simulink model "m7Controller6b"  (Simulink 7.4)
settings: Solver=FixedStepDiscrete  StartTime=0.0  StopTime=100  FixedStep=0.1  RelTol=1e-3
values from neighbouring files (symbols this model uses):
  Link1 = [pi/2, 0, pi/2, 0]    [robot_parameters.m]
  Link2 = [0, 0.404, pi/2, 0]    [robot_parameters.m]
  Link3 = [-pi/2, 0, 0, 0]    [robot_parameters.m]
  Link4 = [pi/2, 0.025, 0, 0.405]    [robot_parameters.m]
  Link5 = [pi/2, 0, pi/2, 0]    [robot_parameters.m]
  Link6 = [0, 0, pi/2, 0]    [robot_parameters.m]
  NoOfLinks = 6    [robot_parameters.m]
libraries: vrlib x3, simulink x2

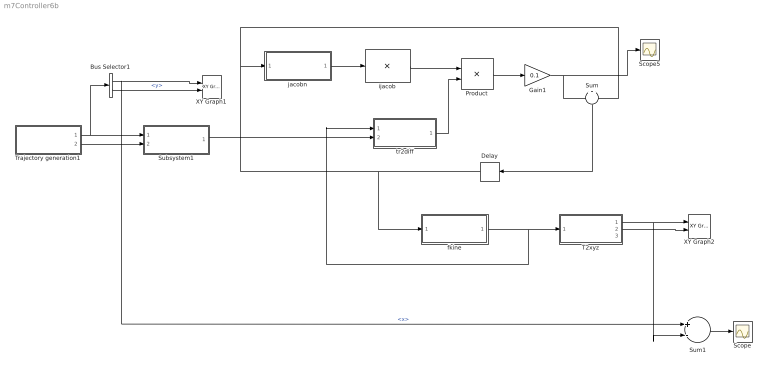
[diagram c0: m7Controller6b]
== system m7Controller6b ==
  Bus Selector1 : BusSelector  OutputSignals=x,y
  Delay : Memory  X0=[pi/2; pi/2; 0; 0; pi/2; pi/2]  InheritSampleTime=on
  Gain1 : Gain  Gain=0.1  ParameterDataType=fixdt(1, 16)  ParameterScaling=2^0  OutDataType=fixdt(1, 16)  OutScaling=2^0
  Product : Product  Multiplication=Matrix(*)  OutDataType=sfix(16)  OutScaling=2^0
  Scope : Scope
  Scope5 : Scope
  Subsystem1 : Subsystem
  Sum : Sum  OutDataType=sfix(16)  OutScaling=2^0
  Sum1 : Sum  Inputs=+-  OutDataType=sfix(16)  OutScaling=2^0
  T2xyz : Subsystem
  Trajectory generation1 : Subsystem
  XY Graph1 : simulink/Sinks/XY Graph  SystemSampleTime=-1  xmin=-0.2  xmax=0.8  ymin=-0.5  ymax=0.5  st=-1
  XY Graph2 : simulink/Sinks/XY Graph  SystemSampleTime=-1  xmin=-0.2  xmax=0.8  ymin=-0.5  ymax=0.5  st=-1
  fkine : Subsystem  TreatAsAtomicUnit=on
  ijacob : Product  Inputs=/  Multiplication=Matrix(*)  OutDataType=fixdt(1, 16)  OutScaling=2^0
  jacobn : Subsystem  TreatAsAtomicUnit=on
  tr2diff : Subsystem
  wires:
  T2xyz/1(x) -> Sum1/2, XY Graph2/1
  fkine/1(T) -> T2xyz/1(T), tr2diff/1(T1)
  jacobn/1(Out1) -> ijacob/1
  ijacob/1 -> Product/1
  Sum/1 -> Delay/1
  Delay/1 -> Sum/2, jacobn/1(q), fkine/1(q)
  Trajectory generation1/1(xyz) -> Subsystem1/1(xyz), Bus Selector1/1
  Trajectory generation1/2(rpy) -> Subsystem1/2(rpy)
  Bus Selector1/1 -> Sum1/1, XY Graph1/1  "<x>"
  Subsystem1/1(T) -> tr2diff/2(T2)
  Product/1 -> Gain1/1
  Gain1/1 -> Scope5/1, Sum/1
  Sum1/1 -> Scope/1
  Bus Selector1/2 -> XY Graph1/2  "<y>"
  T2xyz/2(y) -> XY Graph2/2
  tr2diff/1(dx) -> Product/2

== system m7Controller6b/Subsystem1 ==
  xyz : Inport  OutDataType=fixdt(1, 16)  OutScaling=2^0
  rpy : Inport  Port=2  OutDataType=fixdt(1, 16)  OutScaling=2^0
  Bus Selector : BusSelector  OutputSignals=x,y,z
  Bus Selector1 : BusSelector  OutputSignals=roll,pitch,yaw
  Product : Product  Multiplication=Matrix(*)  OutDataType=fixdt(1, 16)  OutScaling=2^0
  rpy2T : Subsystem
  xyz2T : Subsystem
  T : Outport  OutDataType=fixdt(1, 16)  OutScaling=2^0
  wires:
  xyz/1 -> Bus Selector/1
  Bus Selector/1 -> xyz2T/1(x)  "<x>"
  Bus Selector/2 -> xyz2T/2(y)  "<y>"
  Bus Selector/3 -> xyz2T/3(z)  "<z>"
  xyz2T/1(T) -> Product/1
  Product/1 -> T/1
  rpy2T/1(T) -> Product/2
  rpy/1 -> Bus Selector1/1
  Bus Selector1/1 -> rpy2T/1(roll)  "<roll>"
  Bus Selector1/2 -> rpy2T/2(pitch)  "<pitch>"
  Bus Selector1/3 -> rpy2T/3(yaw)  "<yaw>"

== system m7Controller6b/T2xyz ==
  T : Inport  OutDataType=fixdt(1, 16)  OutScaling=2^0
  Selector : Selector  NumberOfDimensions=2  InputPortWidth=3  IndexOptions=Index vector (dialog),Index vector (dialog)  Indices=1,4  OutputSizes=1,1
  Selector1 : Selector  NumberOfDimensions=2  InputPortWidth=3  IndexOptions=Index vector (dialog),Index vector (dialog)  Indices=2,4  OutputSizes=1,1
  Selector2 : Selector  NumberOfDimensions=2  InputPortWidth=3  IndexOptions=Index vector (dialog),Index vector (dialog)  Indices=3,4  OutputSizes=1,1
  x : Outport  OutDataType=fixdt(1, 16)  OutScaling=2^0
  y : Outport  Port=2  OutDataType=fixdt(1, 16)  OutScaling=2^0
  z : Outport  Port=3  OutDataType=fixdt(1, 16)  OutScaling=2^0
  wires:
  Selector/1 -> x/1
  Selector1/1 -> y/1
  Selector2/1 -> z/1
  T/1 -> Selector/1, Selector2/1, Selector1/1

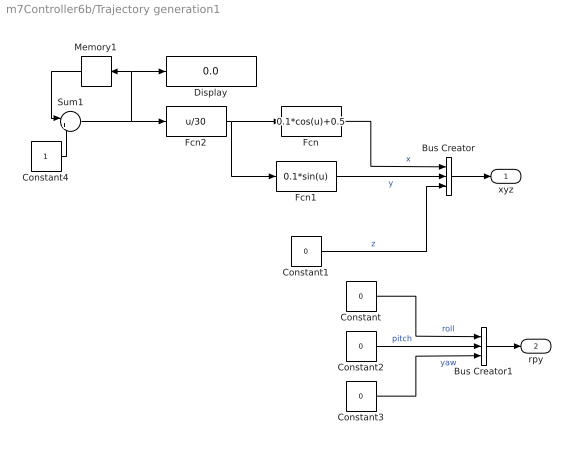
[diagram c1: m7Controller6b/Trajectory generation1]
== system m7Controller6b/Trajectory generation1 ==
  Bus Creator : BusCreator  Inputs='x','y','z'
  Bus Creator1 : BusCreator  Inputs=3
  Constant : Constant  Value=0  VectorParams1D=off  OutDataType=fixdt(1, 16)  OutScaling=2^0
  Constant1 : Constant  Value=0
  Constant2 : Constant  Value=0  OutDataType=fixdt(1, 16)  OutScaling=2^0
  Constant3 : Constant  Value=0  OutDataType=fixdt(1, 16)  OutScaling=2^0
  Constant4 : Constant  OutDataType=fixdt(1, 16)  OutScaling=2^0
  Display : Display
  Fcn : Fcn  Expr=0.1*cos(u)+0.5
  Fcn1 : Fcn  Expr=0.1*sin(u)
  Fcn2 : Fcn  Expr=u/30
  Memory1 : Memory
  Sum1 : Sum  Inputs=|++  OutDataType=sfix(16)  OutScaling=2^0
  xyz : Outport  OutDataType=fixdt(1, 16)  OutScaling=2^0
  rpy : Outport  Port=2  OutDataType=fixdt(1, 16)  OutScaling=2^0
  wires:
  Constant1/1 -> Bus Creator/3  "z"
  Fcn2/1 -> Fcn/1, Fcn1/1
  Fcn/1 -> Bus Creator/1  "x"
  Fcn1/1 -> Bus Creator/2  "y"
  Bus Creator/1 -> xyz/1
  Constant2/1 -> Bus Creator1/2  "pitch"
  Constant/1 -> Bus Creator1/1  "roll"
  Constant3/1 -> Bus Creator1/3  "yaw"
  Bus Creator1/1 -> rpy/1
  Memory1/1 -> Sum1/1
  Sum1/1 -> Fcn2/1, Display/1, Memory1/1
  Constant4/1 -> Sum1/2

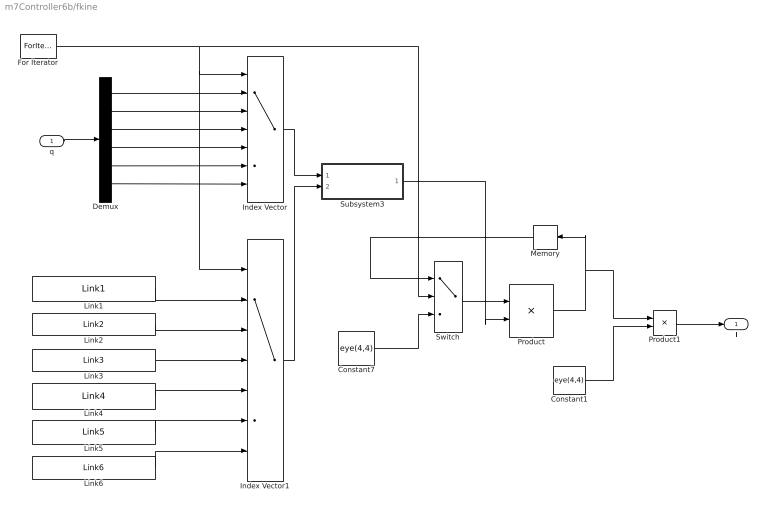
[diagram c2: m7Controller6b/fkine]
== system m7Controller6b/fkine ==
  q : Inport  OutDataType=fixdt(1, 16)  OutScaling=2^0
  Constant1 : Constant  Value=eye(4,4)  OutDataType=fixdt(1, 16)  OutScaling=2^0
  Constant7 : Constant  Value=eye(4,4)  OutDataType=fixdt(1, 16)  OutScaling=2^0
  Demux : Demux  Outputs=6
  For Iterator : ForIterator  IterationLimit=NoOfLinks
  Index Vector : MultiPortSwitch  Inputs=6  OutDataType=fixdt(1, 16)  OutScaling=2^0
  Index Vector1 : MultiPortSwitch  Inputs=6  OutDataType=fixdt(1, 16)  OutScaling=2^0
  Link1 : Constant  Value=Link1  OutDataType=fixdt(1, 16)  OutScaling=2^0
  Link2 : Constant  Value=Link2  OutDataType=fixdt(1, 16)  OutScaling=2^0
  Link3 : Constant  Value=Link3  OutDataType=fixdt(1, 16)  OutScaling=2^0
  Link4 : Constant  Value=Link4  OutDataType=fixdt(1, 16)  OutScaling=2^0
  Link5 : Constant  Value=Link5  OutDataType=fixdt(1, 16)  OutScaling=2^0
  Link6 : Constant  Value=Link6  OutDataType=fixdt(1, 16)  OutScaling=2^0
  Memory : Memory  X0=eye(4,4)  InheritSampleTime=on
  Product : Product  Multiplication=Matrix(*)  OutDataType=fixdt(1, 16)  OutScaling=2^0
  Product1 : Product  Multiplication=Matrix(*)  OutDataType=fixdt(1,8,2)
  Subsystem3 : Subsystem
  Switch : Switch  Criteria=u2 > Threshold  Threshold=1  OutDataType=fixdt(1, 16)  OutScaling=2^0
  T : Outport  OutDataType=fixdt(1, 16)  OutScaling=2^0
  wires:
  Memory/1 -> Switch/1
  Switch/1 -> Product/1
  Subsystem3/1(Out1) -> Product/2
  Constant7/1 -> Switch/3
  Product/1 -> Product1/1, Memory/1
  Index Vector1/1 -> Subsystem3/2(In2)
  Index Vector/1 -> Subsystem3/1(In1)
  Demux/6 -> Index Vector/7
  Demux/5 -> Index Vector/6
  Demux/4 -> Index Vector/5
  Demux/3 -> Index Vector/4
  Demux/2 -> Index Vector/3
  Demux/1 -> Index Vector/2
  q/1 -> Demux/1
  Link6/1 -> Index Vector1/7
  Link5/1 -> Index Vector1/6
  Link4/1 -> Index Vector1/5
  Link3/1 -> Index Vector1/4
  Link2/1 -> Index Vector1/3
  Link1/1 -> Index Vector1/2
  For Iterator/1 -> Switch/2, Index Vector1/1, Index Vector/1
  Product1/1 -> T/1
  Constant1/1 -> Product1/2

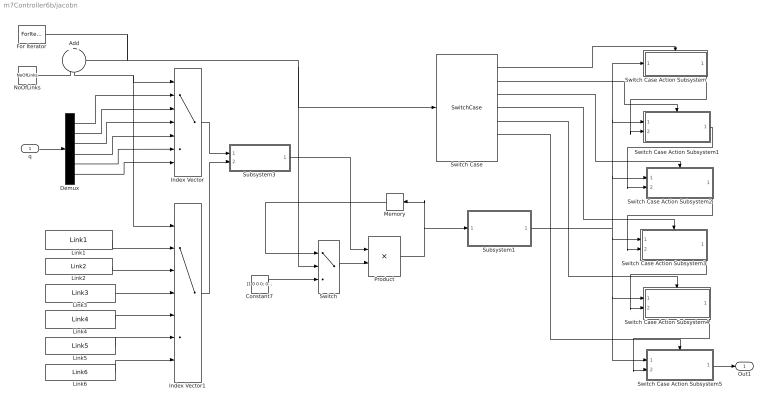
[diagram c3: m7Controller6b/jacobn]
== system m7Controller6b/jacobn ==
  q : Inport  OutDataType=fixdt(1, 16)  OutScaling=2^0
  Add : Sum  Inputs=+-  OutDataType=fixdt(1, 16)  OutScaling=2^-10
  Constant7 : Constant  Value=[1 0 0 0; 0 1 0 0; 0 0 1 0; 0 0 0 1]  OutDataType=fixdt(1, 16)  OutScaling=2^0
  Demux : Demux  Outputs=6
  For Iterator : ForIterator  IterationLimit=NoOfLinks
  Index Vector : MultiPortSwitch  Inputs=6  zeroidx=on  OutDataType=fixdt(1, 16)  OutScaling=2^0
  Index Vector1 : MultiPortSwitch  Inputs=6  zeroidx=on  OutDataType=fixdt(1, 16)  OutScaling=2^0
  Link1 : Constant  Value=Link1  OutDataType=fixdt(1, 16)  OutScaling=2^0
  Link2 : Constant  Value=Link2  OutDataType=fixdt(1, 16)  OutScaling=2^0
  Link3 : Constant  Value=Link3  OutDataType=fixdt(1, 16)  OutScaling=2^0
  Link4 : Constant  Value=Link4  OutDataType=fixdt(1, 16)  OutScaling=2^0
  Link5 : Constant  Value=Link5  OutDataType=fixdt(1, 16)  OutScaling=2^0
  Link6 : Constant  Value=Link6  OutDataType=fixdt(1, 16)  OutScaling=2^0
  Memory : Memory  X0=[1 0 0 0; 0 1 0 0; 0 0 1 0; 0 0 0 1]  InheritSampleTime=on
  NoOfLinks : Constant  Value=NoOfLinks  OutDataType=fixdt(1, 16)  OutScaling=2^0
  Product : Product  Multiplication=Matrix(*)  OutDataType=fixdt(1, 16)  OutScaling=2^0
  Subsystem1 : Subsystem
  Subsystem3 : Subsystem
  Switch : Switch  Threshold=1  OutDataType=fixdt(1, 16)  OutScaling=2^0
  Switch Case : SwitchCase  CaseConditions={1, 2, 3, 4, 5, 6}
  Switch Case Action Subsystem : Subsystem  TreatAsAtomicUnit=on
  Switch Case Action Subsystem1 : Subsystem  TreatAsAtomicUnit=on
  Switch Case Action Subsystem2 : Subsystem  TreatAsAtomicUnit=on
  Switch Case Action Subsystem3 : Subsystem  TreatAsAtomicUnit=on
  Switch Case Action Subsystem4 : Subsystem  TreatAsAtomicUnit=on
  Switch Case Action Subsystem5 : Subsystem  TreatAsAtomicUnit=on
  Out1 : Outport  OutDataType=fixdt(1, 16)  OutScaling=2^0
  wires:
  NoOfLinks/1 -> Add/1
  For Iterator/1 -> Add/2, Switch/2, Switch Case/1
  Add/1 -> Index Vector/1, Index Vector1/1
  Link1/1 -> Index Vector1/2
  Link2/1 -> Index Vector1/3
  Link3/1 -> Index Vector1/4
  Link4/1 -> Index Vector1/5
  Link5/1 -> Index Vector1/6
  Link6/1 -> Index Vector1/7
  q/1 -> Demux/1
  Demux/1 -> Index Vector/2
  Demux/2 -> Index Vector/3
  Demux/3 -> Index Vector/4
  Demux/4 -> Index Vector/5
  Demux/5 -> Index Vector/6
  Demux/6 -> Index Vector/7
  Index Vector/1 -> Subsystem3/1(In1)
  Index Vector1/1 -> Subsystem3/2(In2)
  Product/1 -> Memory/1, Subsystem1/1(In1)
  Constant7/1 -> Switch/3
  Subsystem3/1(Out1) -> Product/1
  Switch/1 -> Product/2
  Memory/1 -> Switch/1
  Subsystem1/1(Out1) -> Switch Case Action Subsystem/1(In1), Switch Case Action Subsystem1/1(In1), Switch Case Action Subsystem2/1(In1), Switch Case Action Subsystem5/1(In1), Switch Case Action Subsystem4/1(In1), Switch Case Action Subsystem3/1(In1)
  Switch Case/1 -> Switch Case Action Subsystem/Action
  Switch Case/2 -> Switch Case Action Subsystem1/Action
  Switch Case/3 -> Switch Case Action Subsystem2/Action
  Switch Case/4 -> Switch Case Action Subsystem3/Action
  Switch Case/5 -> Switch Case Action Subsystem4/Action
  Switch Case/6 -> Switch Case Action Subsystem5/Action
  Switch Case Action Subsystem5/1(Out1) -> Out1/1
  Switch Case Action Subsystem1/1(Out1) -> Switch Case Action Subsystem2/2(In2)
  Switch Case Action Subsystem/1(Out1) -> Switch Case Action Subsystem1/2(In2)
  Switch Case Action Subsystem2/1(Out1) -> Switch Case Action Subsystem3/2(In2)
  Switch Case Action Subsystem3/1(Out1) -> Switch Case Action Subsystem4/2(In2)
  Switch Case Action Subsystem4/1(Out1) -> Switch Case Action Subsystem5/2(In2)

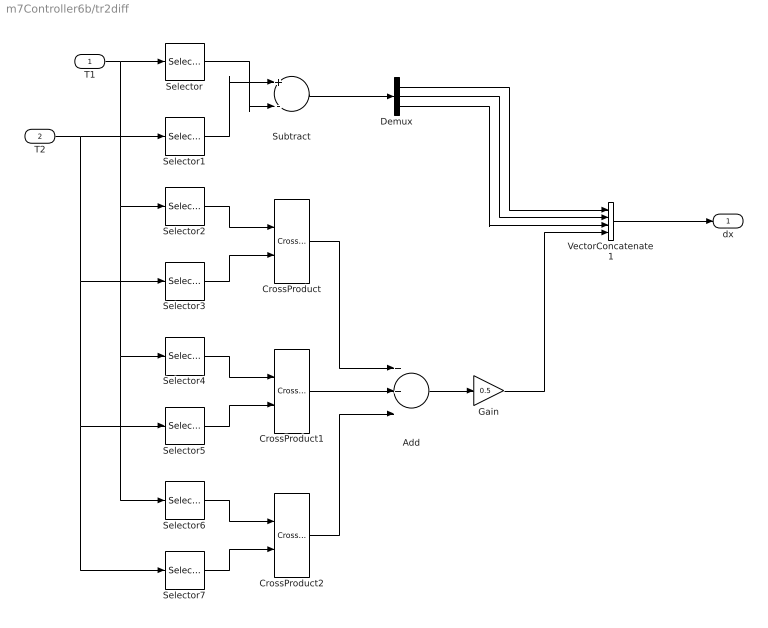
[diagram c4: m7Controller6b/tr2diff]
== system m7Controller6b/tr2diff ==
  T1 : Inport  OutDataType=fixdt(1, 16)  OutScaling=2^0
  T2 : Inport  Port=2  OutDataType=fixdt(1, 16)  OutScaling=2^0
  Add : Sum  Inputs=+++  OutDataType=fixdt(1, 16)  OutScaling=2^-10
  CrossProduct : vrlib/Utilities/Cross Product  SystemSampleTime=-1
  CrossProduct1 : vrlib/Utilities/Cross Product  SystemSampleTime=-1
  CrossProduct2 : vrlib/Utilities/Cross Product  SystemSampleTime=-1
  Demux : Demux  Outputs=3
  Gain : Gain  Gain=0.5  ParameterDataType=fixdt(1, 16)  ParameterScaling=2^0  OutDataType=fixdt(1, 16)  OutScaling=2^0
  Selector : Selector  NumberOfDimensions=2  InputPortWidth=3  IndexOptions=Index vector (dialog),Index vector (dialog)  Indices=[1:3],4  OutputSizes=1,1
  Selector1 : Selector  NumberOfDimensions=2  InputPortWidth=3  IndexOptions=Index vector (dialog),Index vector (dialog)  Indices=[1:3],4  OutputSizes=1,1
  Selector2 : Selector  NumberOfDimensions=2  InputPortWidth=3  IndexOptions=Index vector (dialog),Index vector (dialog)  Indices=[1:3],1  OutputSizes=1,1
  Selector3 : Selector  NumberOfDimensions=2  InputPortWidth=3  IndexOptions=Index vector (dialog),Index vector (dialog)  Indices=[1:3],1  OutputSizes=1,1
  Selector4 : Selector  NumberOfDimensions=2  InputPortWidth=3  IndexOptions=Index vector (dialog),Index vector (dialog)  Indices=[1:3],2  OutputSizes=1,1
  Selector5 : Selector  NumberOfDimensions=2  InputPortWidth=3  IndexOptions=Index vector (dialog),Index vector (dialog)  Indices=[1:3],2  OutputSizes=1,1
  Selector6 : Selector  NumberOfDimensions=2  InputPortWidth=3  IndexOptions=Index vector (dialog),Index vector (dialog)  Indices=[1:3],3  OutputSizes=1,1
  Selector7 : Selector  NumberOfDimensions=2  InputPortWidth=3  IndexOptions=Index vector (dialog),Index vector (dialog)  Indices=[1:3],3  OutputSizes=1,1
  Subtract : Sum  Inputs=+-  OutDataType=fixdt(1, 16)  OutScaling=2^-10
  VectorConcatenate1 : Concatenate  NumInputs=4  Mode=Vector
  dx : Outport  OutDataType=fixdt(1, 16)  OutScaling=2^0
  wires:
  T1/1 -> Selector/1, Selector2/1, Selector6/1, Selector4/1
  T2/1 -> Selector1/1, Selector7/1, Selector5/1, Selector3/1
  Selector1/1 -> Subtract/1
  Selector/1 -> Subtract/2
  Selector2/1 -> CrossProduct/1
  Selector3/1 -> CrossProduct/2
  Selector4/1 -> CrossProduct1/1
  Selector5/1 -> CrossProduct1/2
  Selector6/1 -> CrossProduct2/1
  Selector7/1 -> CrossProduct2/2
  CrossProduct/1 -> Add/1
  CrossProduct1/1 -> Add/2
  CrossProduct2/1 -> Add/3
  Add/1 -> Gain/1
  VectorConcatenate1/1 -> dx/1
  Subtract/1 -> Demux/1
  Demux/1 -> VectorConcatenate1/1
  Demux/2 -> VectorConcatenate1/2
  Demux/3 -> VectorConcatenate1/3
  Gain/1 -> VectorConcatenate1/4

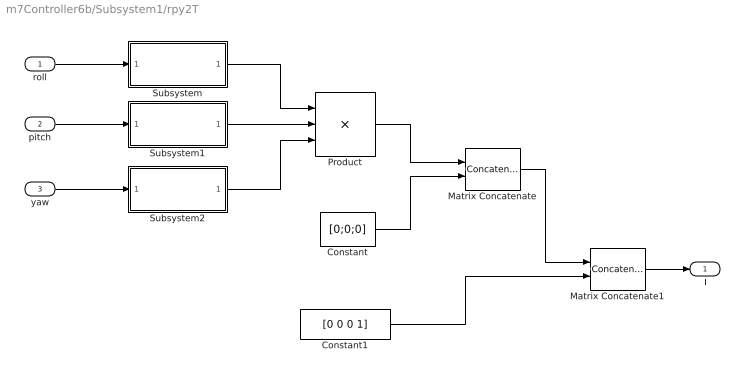
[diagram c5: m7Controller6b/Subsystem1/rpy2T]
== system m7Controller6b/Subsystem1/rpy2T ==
  roll : Inport  OutDataType=fixdt(1, 16)  OutScaling=2^0
  pitch : Inport  Port=2  OutDataType=fixdt(1, 16)  OutScaling=2^0
  yaw : Inport  Port=3  OutDataType=fixdt(1, 16)  OutScaling=2^0
  Constant : Constant  Value=[0;0;0]  OutDataType=fixdt(1, 16)  OutScaling=2^0
  Constant1 : Constant  Value=[0 0 0 1]  VectorParams1D=off  OutDataType=fixdt(1, 16)  OutScaling=2^0
  Matrix Concatenate : Concatenate  Mode=Multidimensional array  ConcatenateDimension=2
  Matrix Concatenate1 : Concatenate  Mode=Multidimensional array
  Product : Product  Inputs=3  Multiplication=Matrix(*)  OutDataType=fixdt(1, 16)  OutScaling=2^0
  Subsystem : Subsystem
  Subsystem1 : Subsystem
  Subsystem2 : Subsystem
  T : Outport  OutDataType=fixdt(1, 16)  OutScaling=2^0
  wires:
  roll/1 -> Subsystem/1(roll)
  pitch/1 -> Subsystem1/1(roll)
  yaw/1 -> Subsystem2/1(roll)
  Subsystem/1(Out1) -> Product/1
  Subsystem1/1(Out1) -> Product/2
  Subsystem2/1(Out1) -> Product/3
  Product/1 -> Matrix Concatenate/1
  Constant/1 -> Matrix Concatenate/2
  Matrix Concatenate/1 -> Matrix Concatenate1/1
  Constant1/1 -> Matrix Concatenate1/2
  Matrix Concatenate1/1 -> T/1

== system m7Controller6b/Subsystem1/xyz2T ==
  x : Inport  OutDataType=fixdt(1, 16)  OutScaling=2^0
  y : Inport  Port=2  OutDataType=fixdt(1, 16)  OutScaling=2^0
  z : Inport  Port=3  OutDataType=fixdt(1, 16)  OutScaling=2^0
  Constant : Constant  Value=eye(3)  OutDataType=fixdt(1, 16)  OutScaling=2^0
  Constant1 : Constant  Value=[0 0 0 1]  VectorParams1D=off  OutDataType=fixdt(1, 16)  OutScaling=2^0
  Matrix Concatenate : Concatenate  Mode=Multidimensional array  ConcatenateDimension=2
  Matrix Concatenate1 : Concatenate  Mode=Multidimensional array
  Vector Concatenate : Concatenate  NumInputs=3  Mode=Vector
  T : Outport  OutDataType=fixdt(1, 16)  OutScaling=2^0
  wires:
  x/1 -> Vector Concatenate/1
  y/1 -> Vector Concatenate/2
  z/1 -> Vector Concatenate/3
  Constant/1 -> Matrix Concatenate/1
  Vector Concatenate/1 -> Matrix Concatenate/2
  Matrix Concatenate/1 -> Matrix Concatenate1/1
  Constant1/1 -> Matrix Concatenate1/2
  Matrix Concatenate1/1 -> T/1

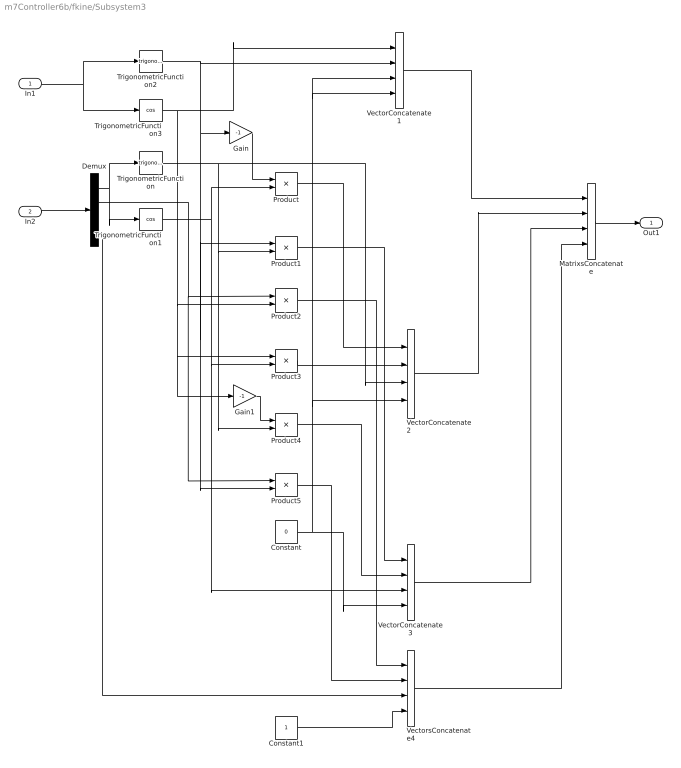
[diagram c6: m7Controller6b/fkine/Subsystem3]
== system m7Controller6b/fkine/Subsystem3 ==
  In1 : Inport  OutDataType=fixdt(1, 16)  OutScaling=2^0
  In2 : Inport  Port=2  OutDataType=fixdt(1, 16)  OutScaling=2^0
  Constant : Constant  Value=0  OutDataType=fixdt(1, 16)  OutScaling=2^0
  Constant1 : Constant  OutDataType=fixdt(1, 16)  OutScaling=2^0
  Demux : Demux
  Gain : Gain  Gain=-1  ParameterDataType=fixdt(1, 16)  ParameterScaling=2^0  OutDataType=fixdt(1, 16)  OutScaling=2^0
  Gain1 : Gain  Gain=-1  ParameterDataType=fixdt(1, 16)  ParameterScaling=2^0  OutDataType=fixdt(1, 16)  OutScaling=2^0
  MatrixsConcatenate : Concatenate  NumInputs=4  Mode=Multidimensional array  ConcatenateDimension=2
  Product{,1..5} (6 alike) : Product  OutDataType=fixdt(1, 16)  OutScaling=2^0
  TrigonometricFunction : Trigonometry
  TrigonometricFunction1 : Trigonometry  Operator=cos
  TrigonometricFunction2 : Trigonometry
  TrigonometricFunction3 : Trigonometry  Operator=cos
  VectorConcatenate1 : Concatenate  NumInputs=4  Mode=Vector  ConcatenateDimension=2
  VectorConcatenate2 : Concatenate  NumInputs=4  Mode=Vector  ConcatenateDimension=2
  VectorConcatenate3 : Concatenate  NumInputs=4  Mode=Vector  ConcatenateDimension=2
  VectorsConcatenate4 : Concatenate  NumInputs=4  Mode=Vector  ConcatenateDimension=2
  Out1 : Outport  OutDataType=fixdt(1, 16)  OutScaling=2^0
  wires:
  VectorsConcatenate4/1 -> MatrixsConcatenate/4
  VectorConcatenate3/1 -> MatrixsConcatenate/3
  VectorConcatenate2/1 -> MatrixsConcatenate/2
  VectorConcatenate1/1 -> MatrixsConcatenate/1
  MatrixsConcatenate/1 -> Out1/1
  Constant1/1 -> VectorsConcatenate4/4
  Constant/1 -> VectorConcatenate1/3, VectorConcatenate1/4, VectorConcatenate2/4, VectorConcatenate3/4
  Gain1/1 -> Product4/1
  Product3/1 -> VectorConcatenate2/2
  Demux/2 -> Product5/1, Product2/1
  TrigonometricFunction/1 -> Product1/2, Product4/2, VectorConcatenate2/3
  TrigonometricFunction3/1 -> VectorConcatenate1/1, Gain1/1, Product3/1, Product2/2
  TrigonometricFunction1/1 -> VectorConcatenate3/3, Product3/2, Product/2
  Gain/1 -> Product/1
  TrigonometricFunction2/1 -> Product1/1, Product5/2, Gain/1, VectorConcatenate1/2
  Demux/1 -> TrigonometricFunction1/1, TrigonometricFunction/1
  In1/1 -> TrigonometricFunction3/1, TrigonometricFunction2/1
  In2/1 -> Demux/1
  Product/1 -> VectorConcatenate2/1
  Product4/1 -> VectorConcatenate3/2
  Product1/1 -> VectorConcatenate3/1
  Product2/1 -> VectorsConcatenate4/1
  Product5/1 -> VectorsConcatenate4/2
  Demux/4 -> VectorsConcatenate4/3

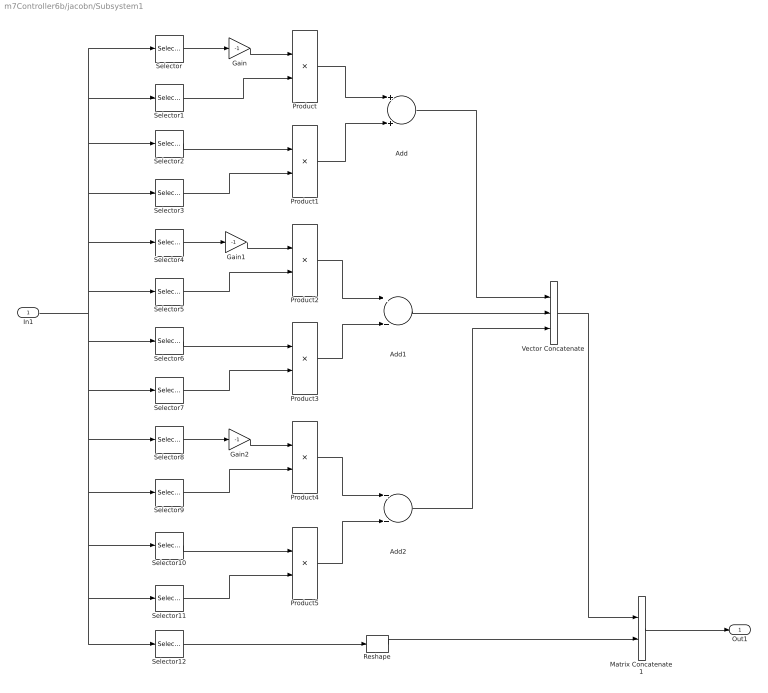
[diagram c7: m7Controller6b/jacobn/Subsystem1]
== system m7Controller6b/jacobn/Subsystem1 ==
  In1 : Inport
  Add : Sum  OutDataType=fixdt(1, 16)  OutScaling=2^-10
  Add1 : Sum  OutDataType=fixdt(1, 16)  OutScaling=2^-10
  Add2 : Sum  OutDataType=fixdt(1, 16)  OutScaling=2^-10
  Gain : Gain  Gain=-1  ParameterDataType=fixdt(1, 16)  ParameterScaling=2^0  OutDataType=fixdt(1, 16)  OutScaling=2^0
  Gain1 : Gain  Gain=-1  ParameterDataType=fixdt(1, 16)  ParameterScaling=2^0  OutDataType=fixdt(1, 16)  OutScaling=2^0
  Gain2 : Gain  Gain=-1  ParameterDataType=fixdt(1, 16)  ParameterScaling=2^0  OutDataType=fixdt(1, 16)  OutScaling=2^0
  Matrix Concatenate1 : Concatenate  Mode=Multidimensional array
  Product{,1..5} (6 alike) : Product  OutDataType=fixdt(1, 16)  OutScaling=2^0
  Reshape : Reshape  OutputDimensionality=Customize  OutputDimensions=[3,1]
  Selector : Selector  NumberOfDimensions=2  InputPortWidth=3  IndexOptions=Index vector (dialog),Index vector (dialog)  Indices=1,1  OutputSizes=1,1
  Selector1 : Selector  NumberOfDimensions=2  InputPortWidth=3  IndexOptions=Index vector (dialog),Index vector (dialog)  Indices=2,4  OutputSizes=1,1
  Selector10 : Selector  NumberOfDimensions=2  InputPortWidth=3  IndexOptions=Index vector (dialog),Index vector (dialog)  Indices=2,3  OutputSizes=1,1
  Selector11 : Selector  NumberOfDimensions=2  InputPortWidth=3  IndexOptions=Index vector (dialog),Index vector (dialog)  Indices=1,4  OutputSizes=1,1
  Selector12 : Selector  NumberOfDimensions=2  InputPortWidth=3  IndexOptions=Index vector (dialog),Index vector (dialog)  Indices=3,[1:3]  OutputSizes=1,1
  Selector2 : Selector  NumberOfDimensions=2  InputPortWidth=3  IndexOptions=Index vector (dialog),Index vector (dialog)  Indices=2,1  OutputSizes=1,1
  Selector3 : Selector  NumberOfDimensions=2  InputPortWidth=3  IndexOptions=Index vector (dialog),Index vector (dialog)  Indices=1,4  OutputSizes=1,1
  Selector4 : Selector  NumberOfDimensions=2  InputPortWidth=3  IndexOptions=Index vector (dialog),Index vector (dialog)  Indices=1,2  OutputSizes=1,1
  Selector5 : Selector  NumberOfDimensions=2  InputPortWidth=3  IndexOptions=Index vector (dialog),Index vector (dialog)  Indices=2,4  OutputSizes=1,1
  Selector6 : Selector  NumberOfDimensions=2  InputPortWidth=3  IndexOptions=Index vector (dialog),Index vector (dialog)  Indices=2,2  OutputSizes=1,1
  Selector7 : Selector  NumberOfDimensions=2  InputPortWidth=3  IndexOptions=Index vector (dialog),Index vector (dialog)  Indices=1,4  OutputSizes=1,1
  Selector8 : Selector  NumberOfDimensions=2  InputPortWidth=3  IndexOptions=Index vector (dialog),Index vector (dialog)  Indices=1,3  OutputSizes=1,1
  Selector9 : Selector  NumberOfDimensions=2  InputPortWidth=3  IndexOptions=Index vector (dialog),Index vector (dialog)  Indices=2,4  OutputSizes=1,1
  Vector Concatenate : Concatenate  NumInputs=3  Mode=Vector
  Out1 : Outport
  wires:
  Selector/1 -> Gain/1
  In1/1 -> Selector/1, Selector1/1, Selector2/1, Selector3/1, Selector4/1, Selector5/1, Selector10/1, Selector11/1, Selector12/1, Selector9/1, Selector8/1, Selector7/1, Selector6/1
  Gain/1 -> Product/1
  Selector1/1 -> Product/2
  Selector2/1 -> Product1/1
  Selector3/1 -> Product1/2
  Selector4/1 -> Gain1/1
  Gain1/1 -> Product2/1
  Selector5/1 -> Product2/2
  Selector6/1 -> Product3/1
  Selector7/1 -> Product3/2
  Selector8/1 -> Gain2/1
  Gain2/1 -> Product4/1
  Selector9/1 -> Product4/2
  Selector10/1 -> Product5/1
  Selector11/1 -> Product5/2
  Product/1 -> Add/1
  Product1/1 -> Add/2
  Product2/1 -> Add1/1
  Product3/1 -> Add1/2
  Product4/1 -> Add2/1
  Product5/1 -> Add2/2
  Add/1 -> Vector Concatenate/1
  Add1/1 -> Vector Concatenate/2
  Add2/1 -> Vector Concatenate/3
  Vector Concatenate/1 -> Matrix Concatenate1/1
  Selector12/1 -> Reshape/1
  Matrix Concatenate1/1 -> Out1/1
  Reshape/1 -> Matrix Concatenate1/2

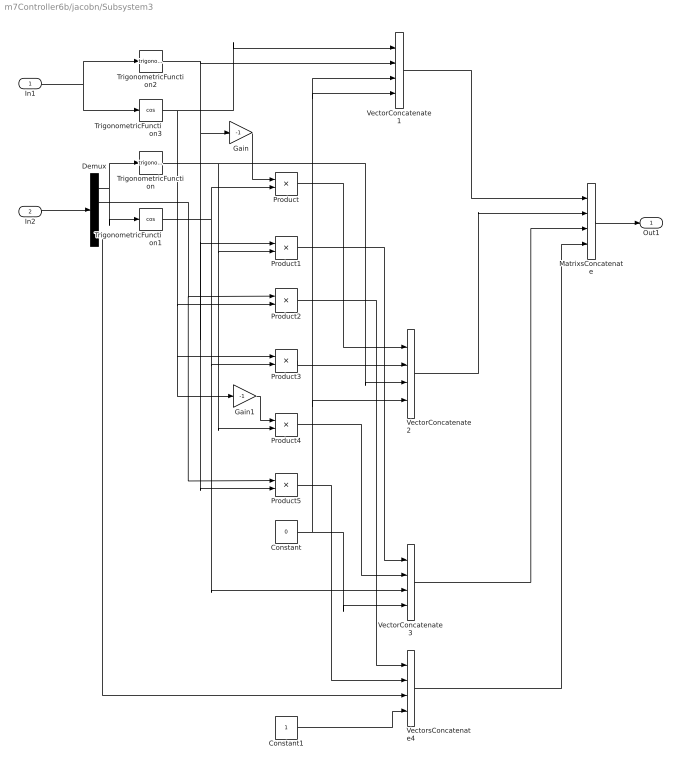
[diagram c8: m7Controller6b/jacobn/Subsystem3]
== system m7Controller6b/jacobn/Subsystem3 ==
  In1 : Inport  OutDataType=fixdt(1, 16)  OutScaling=2^0
  In2 : Inport  Port=2  OutDataType=fixdt(1, 16)  OutScaling=2^0
  Constant : Constant  Value=0  OutDataType=fixdt(1, 16)  OutScaling=2^0
  Constant1 : Constant  OutDataType=fixdt(1, 16)  OutScaling=2^0
  Demux : Demux
  Gain : Gain  Gain=-1  ParameterDataType=fixdt(1, 16)  ParameterScaling=2^0  OutDataType=fixdt(1, 16)  OutScaling=2^0
  Gain1 : Gain  Gain=-1  ParameterDataType=fixdt(1, 16)  ParameterScaling=2^0  OutDataType=fixdt(1, 16)  OutScaling=2^0
  MatrixsConcatenate : Concatenate  NumInputs=4  Mode=Multidimensional array  ConcatenateDimension=2
  Product{,1..5} (6 alike) : Product  OutDataType=fixdt(1, 16)  OutScaling=2^0
  TrigonometricFunction : Trigonometry
  TrigonometricFunction1 : Trigonometry  Operator=cos
  TrigonometricFunction2 : Trigonometry
  TrigonometricFunction3 : Trigonometry  Operator=cos
  VectorConcatenate1 : Concatenate  NumInputs=4  Mode=Vector  ConcatenateDimension=2
  VectorConcatenate2 : Concatenate  NumInputs=4  Mode=Vector  ConcatenateDimension=2
  VectorConcatenate3 : Concatenate  NumInputs=4  Mode=Vector  ConcatenateDimension=2
  VectorsConcatenate4 : Concatenate  NumInputs=4  Mode=Vector  ConcatenateDimension=2
  Out1 : Outport  OutDataType=fixdt(1, 16)  OutScaling=2^0
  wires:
  VectorsConcatenate4/1 -> MatrixsConcatenate/4
  VectorConcatenate3/1 -> MatrixsConcatenate/3
  VectorConcatenate2/1 -> MatrixsConcatenate/2
  VectorConcatenate1/1 -> MatrixsConcatenate/1
  MatrixsConcatenate/1 -> Out1/1
  Constant1/1 -> VectorsConcatenate4/4
  Constant/1 -> VectorConcatenate1/3, VectorConcatenate1/4, VectorConcatenate2/4, VectorConcatenate3/4
  Gain1/1 -> Product4/1
  Product3/1 -> VectorConcatenate2/2
  Demux/2 -> Product5/1, Product2/1
  TrigonometricFunction/1 -> Product1/2, Product4/2, VectorConcatenate2/3
  TrigonometricFunction3/1 -> VectorConcatenate1/1, Gain1/1, Product3/1, Product2/2
  TrigonometricFunction1/1 -> VectorConcatenate3/3, Product3/2, Product/2
  Gain/1 -> Product/1
  TrigonometricFunction2/1 -> Product1/1, Product5/2, Gain/1, VectorConcatenate1/2
  Demux/1 -> TrigonometricFunction1/1, TrigonometricFunction/1
  In1/1 -> TrigonometricFunction3/1, TrigonometricFunction2/1
  In2/1 -> Demux/1
  Product/1 -> VectorConcatenate2/1
  Product4/1 -> VectorConcatenate3/2
  Product1/1 -> VectorConcatenate3/1
  Product2/1 -> VectorsConcatenate4/1
  Product5/1 -> VectorsConcatenate4/2
  Demux/4 -> VectorsConcatenate4/3

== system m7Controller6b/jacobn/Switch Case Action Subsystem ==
  In1 : Inport  OutDataType=fixdt(1, 16)  OutScaling=2^0
  Action Port : ActionPort  ActionType=case
  Matrix Concatenate : Concatenate  NumInputs=1  Mode=Multidimensional array  ConcatenateDimension=2
  Out1 : Outport  OutDataType=fixdt(1, 16)  OutScaling=2^0
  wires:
  In1/1 -> Matrix Concatenate/1
  Matrix Concatenate/1 -> Out1/1

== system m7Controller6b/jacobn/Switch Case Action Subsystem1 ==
  In1 : Inport  OutDataType=fixdt(1, 16)  OutScaling=2^0
  In2 : Inport  Port=2  OutDataType=fixdt(1, 16)  OutScaling=2^0
  Action Port : ActionPort  ActionType=case
  Matrix Concatenate : Concatenate  Mode=Multidimensional array  ConcatenateDimension=2
  Out1 : Outport  OutDataType=fixdt(1, 16)  OutScaling=2^0
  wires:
  In1/1 -> Matrix Concatenate/1
  In2/1 -> Matrix Concatenate/2
  Matrix Concatenate/1 -> Out1/1

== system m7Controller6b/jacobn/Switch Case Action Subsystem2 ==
  In1 : Inport  OutDataType=fixdt(1, 16)  OutScaling=2^0
  In2 : Inport  Port=2  OutDataType=fixdt(1, 16)  OutScaling=2^0
  Action Port : ActionPort  ActionType=case
  Matrix Concatenate : Concatenate  Mode=Multidimensional array  ConcatenateDimension=2
  Out1 : Outport  OutDataType=fixdt(1, 16)  OutScaling=2^0
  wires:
  Matrix Concatenate/1 -> Out1/1
  In2/1 -> Matrix Concatenate/2
  In1/1 -> Matrix Concatenate/1

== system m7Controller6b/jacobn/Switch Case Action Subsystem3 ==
  In1 : Inport  OutDataType=fixdt(1, 16)  OutScaling=2^0
  In2 : Inport  Port=2  OutDataType=fixdt(1, 16)  OutScaling=2^0
  Action Port : ActionPort  ActionType=case
  Matrix Concatenate : Concatenate  Mode=Multidimensional array  ConcatenateDimension=2
  Out1 : Outport  OutDataType=fixdt(1, 16)  OutScaling=2^0
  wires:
  In1/1 -> Matrix Concatenate/1
  In2/1 -> Matrix Concatenate/2
  Matrix Concatenate/1 -> Out1/1

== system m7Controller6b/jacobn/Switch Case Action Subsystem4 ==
  In1 : Inport  OutDataType=fixdt(1, 16)  OutScaling=2^0
  In2 : Inport  Port=2  OutDataType=fixdt(1, 16)  OutScaling=2^0
  Action Port : ActionPort  ActionType=case
  Matrix Concatenate : Concatenate  Mode=Multidimensional array  ConcatenateDimension=2
  Out1 : Outport  OutDataType=fixdt(1, 16)  OutScaling=2^0
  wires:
  Matrix Concatenate/1 -> Out1/1
  In2/1 -> Matrix Concatenate/2
  In1/1 -> Matrix Concatenate/1

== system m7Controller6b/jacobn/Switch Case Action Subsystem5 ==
  In1 : Inport  OutDataType=fixdt(1, 16)  OutScaling=2^0
  In2 : Inport  Port=2  OutDataType=fixdt(1, 16)  OutScaling=2^0
  Action Port : ActionPort  ActionType=case
  Matrix Concatenate : Concatenate  Mode=Multidimensional array  ConcatenateDimension=2
  Out1 : Outport  OutDataType=fixdt(1, 16)  OutScaling=2^0
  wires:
  In1/1 -> Matrix Concatenate/1
  In2/1 -> Matrix Concatenate/2
  Matrix Concatenate/1 -> Out1/1

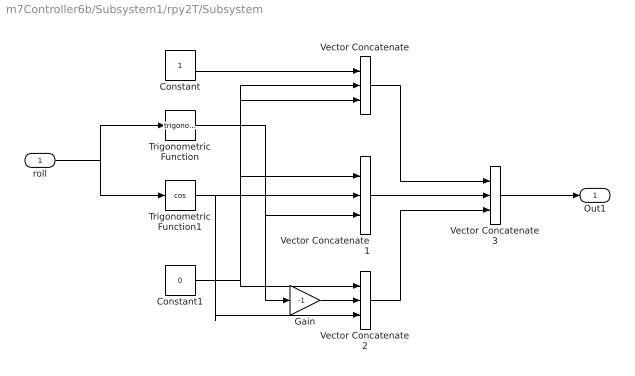
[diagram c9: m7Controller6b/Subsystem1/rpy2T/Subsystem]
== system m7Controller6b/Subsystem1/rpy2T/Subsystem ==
  roll : Inport  OutDataType=fixdt(1, 16)  OutScaling=2^0
  Constant : Constant  OutDataType=fixdt(1, 16)  OutScaling=2^0
  Constant1 : Constant  Value=0  OutDataType=fixdt(1, 16)  OutScaling=2^0
  Gain : Gain  Gain=-1  ParameterDataType=fixdt(1, 16)  ParameterScaling=2^0  OutDataType=fixdt(1, 16)  OutScaling=2^0
  Trigonometric Function : Trigonometry
  Trigonometric Function1 : Trigonometry  Operator=cos
  Vector Concatenate : Concatenate  NumInputs=3  Mode=Vector
  Vector Concatenate1 : Concatenate  NumInputs=3  Mode=Vector
  Vector Concatenate2 : Concatenate  NumInputs=3  Mode=Vector
  Vector Concatenate3 : Concatenate  NumInputs=3  Mode=Multidimensional array  ConcatenateDimension=2
  Out1 : Outport  OutDataType=fixdt(1, 16)  OutScaling=2^0
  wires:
  roll/1 -> Trigonometric Function/1, Trigonometric Function1/1
  Constant/1 -> Vector Concatenate/1
  Trigonometric Function1/1 -> Vector Concatenate1/2, Vector Concatenate2/3
  Trigonometric Function/1 -> Gain/1, Vector Concatenate1/3
  Vector Concatenate/1 -> Vector Concatenate3/1
  Vector Concatenate1/1 -> Vector Concatenate3/2
  Vector Concatenate2/1 -> Vector Concatenate3/3
  Constant1/1 -> Vector Concatenate/2, Vector Concatenate/3, Vector Concatenate1/1, Vector Concatenate2/1
  Gain/1 -> Vector Concatenate2/2
  Vector Concatenate3/1 -> Out1/1

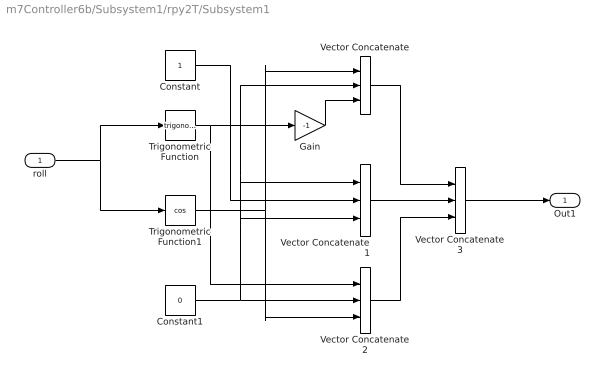
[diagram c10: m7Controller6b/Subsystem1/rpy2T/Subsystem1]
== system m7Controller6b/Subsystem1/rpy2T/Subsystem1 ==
  roll : Inport  OutDataType=fixdt(1, 16)  OutScaling=2^0
  Constant : Constant  OutDataType=fixdt(1, 16)  OutScaling=2^0
  Constant1 : Constant  Value=0  OutDataType=fixdt(1, 16)  OutScaling=2^0
  Gain : Gain  Gain=-1  ParameterDataType=fixdt(1, 16)  ParameterScaling=2^0  OutDataType=fixdt(1, 16)  OutScaling=2^0
  Trigonometric Function : Trigonometry
  Trigonometric Function1 : Trigonometry  Operator=cos
  Vector Concatenate : Concatenate  NumInputs=3  Mode=Vector
  Vector Concatenate1 : Concatenate  NumInputs=3  Mode=Vector
  Vector Concatenate2 : Concatenate  NumInputs=3  Mode=Vector
  Vector Concatenate3 : Concatenate  NumInputs=3  Mode=Multidimensional array  ConcatenateDimension=2
  Out1 : Outport  OutDataType=fixdt(1, 16)  OutScaling=2^0
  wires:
  roll/1 -> Trigonometric Function/1, Trigonometric Function1/1
  Vector Concatenate/1 -> Vector Concatenate3/1
  Vector Concatenate1/1 -> Vector Concatenate3/2
  Vector Concatenate2/1 -> Vector Concatenate3/3
  Trigonometric Function1/1 -> Vector Concatenate/1, Vector Concatenate2/3
  Constant1/1 -> Vector Concatenate2/2, Vector Concatenate/2, Vector Concatenate1/1, Vector Concatenate1/3
  Trigonometric Function/1 -> Gain/1, Vector Concatenate2/1
  Constant/1 -> Vector Concatenate1/2
  Gain/1 -> Vector Concatenate/3
  Vector Concatenate3/1 -> Out1/1

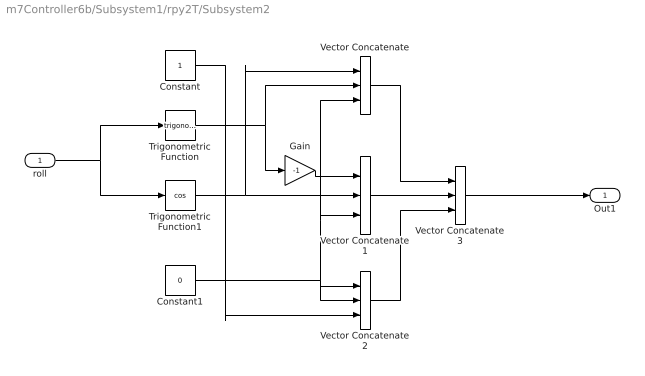
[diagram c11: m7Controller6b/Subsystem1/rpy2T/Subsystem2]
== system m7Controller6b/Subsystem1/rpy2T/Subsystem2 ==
  roll : Inport  OutDataType=fixdt(1, 16)  OutScaling=2^0
  Constant : Constant  OutDataType=fixdt(1, 16)  OutScaling=2^0
  Constant1 : Constant  Value=0  OutDataType=fixdt(1, 16)  OutScaling=2^0
  Gain : Gain  Gain=-1  ParameterDataType=fixdt(1, 16)  ParameterScaling=2^0  OutDataType=fixdt(1, 16)  OutScaling=2^0
  Trigonometric Function : Trigonometry
  Trigonometric Function1 : Trigonometry  Operator=cos
  Vector Concatenate : Concatenate  NumInputs=3  Mode=Vector
  Vector Concatenate1 : Concatenate  NumInputs=3  Mode=Vector
  Vector Concatenate2 : Concatenate  NumInputs=3  Mode=Vector
  Vector Concatenate3 : Concatenate  NumInputs=3  Mode=Multidimensional array  ConcatenateDimension=2
  Out1 : Outport  OutDataType=fixdt(1, 16)  OutScaling=2^0
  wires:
  roll/1 -> Trigonometric Function/1, Trigonometric Function1/1
  Vector Concatenate/1 -> Vector Concatenate3/1
  Vector Concatenate1/1 -> Vector Concatenate3/2
  Vector Concatenate2/1 -> Vector Concatenate3/3
  Trigonometric Function1/1 -> Vector Concatenate/1, Vector Concatenate1/2
  Trigonometric Function/1 -> Vector Concatenate/2, Gain/1
  Constant1/1 -> Vector Concatenate/3, Vector Concatenate1/3, Vector Concatenate2/1, Vector Concatenate2/2
  Constant/1 -> Vector Concatenate2/3
  Gain/1 -> Vector Concatenate1/1
  Vector Concatenate3/1 -> Out1/1
